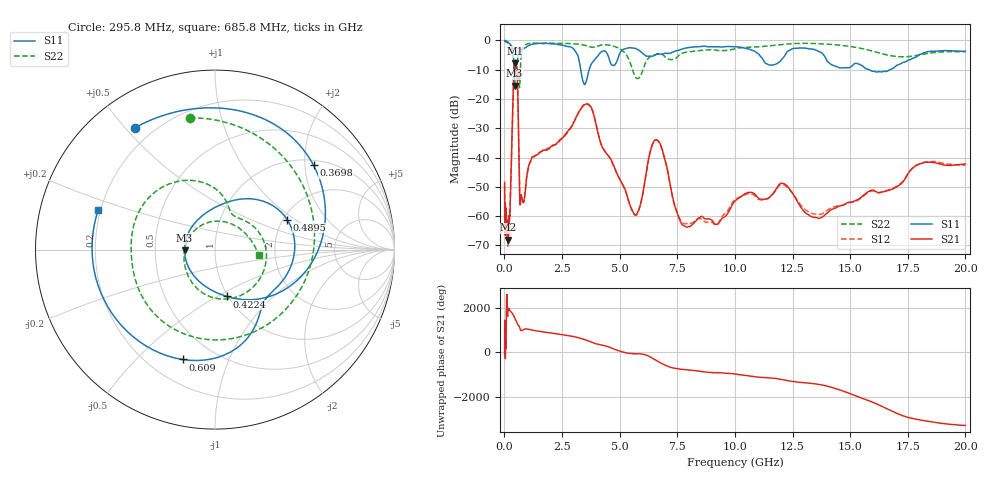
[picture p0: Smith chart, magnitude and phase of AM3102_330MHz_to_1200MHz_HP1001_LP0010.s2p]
! Date/Time: Tue, Sep 11, 2018 5:17 PM
! Network Analyzer: Agilent Technologies E8362B Rev: A.07.50.63
! Sweep from 0.010 to 20.000 GHz, 1601 Points, Sweep Type: LOG
! Power Supply: 4.949 V, 0.001 A
# Hz S DB R 50
!freq MagS11 AngS11 MagS21 AngS21 MagS12 AngS12 MagS22 AngS22
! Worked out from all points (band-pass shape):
!   1601 points, 10 MHz to 20 GHz, reference 50 ohm
!   highest |S21| = -7.78 dB at 460.1 MHz (marker M1); lowest = -68.1 dB at 170.5 MHz (marker M2)
!   |S21| within 3 dB of the highest: 414.3 MHz to 553.7 MHz (139.4 MHz wide, 28.8 % of centre)
!   lowest |S11| = -15.4 dB at 440.9 MHz (marker M3), VSWR 1.41, Z = 35.5 - j0.288 ohm
!   |S11| at or under -10 dB: 418.7 MHz to 467.1 MHz (48.36 MHz wide, 10.9 % of centre); 3.314 GHz to 3.676 GHz (361.8 MHz wide, 10.4 % of centre); 15.84 GHz to 16.72 GHz (886.7 MHz wide, 5.45 % of centre)
!   |S22| runs from -16.2 to -0.2 dB; largest |S21 - S12| = 0.0062
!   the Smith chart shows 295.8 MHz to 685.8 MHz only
!   S11 on the Smith chart (normalised r, x): 295.8 MHz: 0.13, +0.53; 369.8 MHz: 1.13, +2.22; 422.4 MHz: 0.99, -0.56; 489.5 MHz: 2.10, +0.87; 609 MHz: 0.33, -0.69; 685.8 MHz: 0.19, +0.16
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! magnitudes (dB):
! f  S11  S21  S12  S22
! 10 MHz  0.0  -48.4  -49.5  -0.2
! 35.55 MHz  0.0  -63.3  -65.5  -0.3
! 126.4 MHz  -0.4  -65.2  -63.4  -0.7
! 170.5 MHz  -0.6  -68.1  -68.1  -1.0
! 295.8 MHz  -1.8  -43.3  -43.7  -2.5
! 369.8 MHz  -2.8  -20.9  -21.0  -5.7
! 422.4 MHz  -11.4  -9.6  -9.7  -6.3
! 440.9 MHz  -15.4  -8.2  -8.2  -6.6
! 447.2 MHz  -15.1  -7.9  -8.0  -6.6
! 460.1 MHz  -12.0  -7.8  -7.8  -6.5
! 489.5 MHz  -7.2  -8.0  -8.0  -6.9
! 553.8 MHz  -7.7  -10.8  -10.8  -13.3
! 609 MHz  -3.9  -28.6  -28.7  -10.7
! 685.8 MHz  -3.3  -56.1  -56.0  -12.1
! 1.59 GHz  -1.0  -37.9  -37.9  -0.9
! 3.634 GHz  -11.3  -21.9  -21.7  -2.0
! 5.652 GHz  -2.7  -59.5  -59.5  -12.1
! 6.58 GHz  -4.8  -33.9  -34.1  -4.8
! 7.92 GHz  -2.5  -63.8  -62.5  -4.0
! 12.03 GHz  -6.5  -48.7  -49.2  -1.4
! 13.68 GHz  -3.9  -60.7  -59.4  -1.1
! 20 GHz  -3.6  -42.1  -42.6  -3.8
